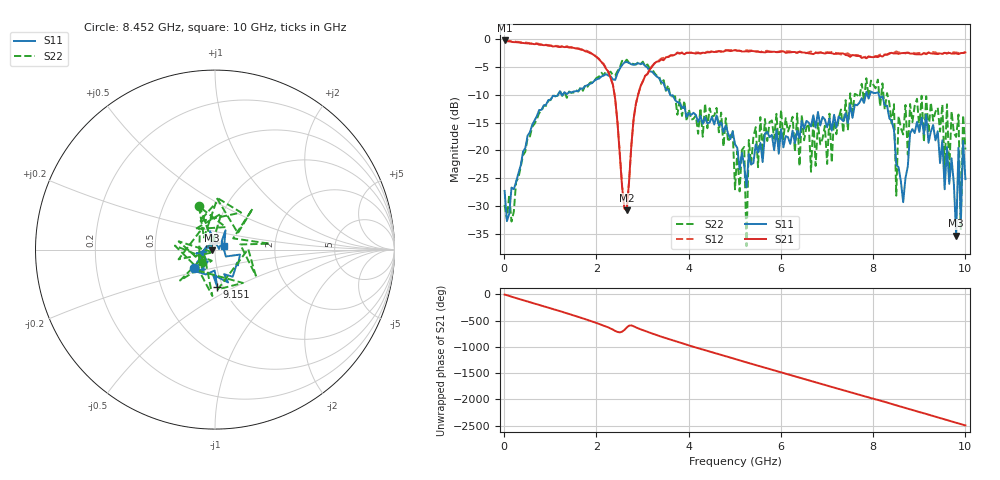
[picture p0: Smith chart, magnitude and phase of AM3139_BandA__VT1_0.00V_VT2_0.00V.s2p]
! Date/Time: Tue, Nov 13, 2018 4:56 PM
! Network Analyzer: Agilent Technologies E8364B Rev: A.07.50.67
! Sweep from 0.010 to 10.000 GHz, 201 Points, Sweep Type: LIN
! Power Supply: -0.000 V, 0.000 A
# Hz S DB R 50
!freq MagS11 AngS11 MagS21 AngS21 MagS12 AngS12 MagS22 AngS22
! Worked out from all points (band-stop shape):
!   201 points, 10 MHz to 10 GHz, reference 50 ohm
!   highest |S21| = -0.20 dB at 10 MHz (marker M1); lowest = -30.8 dB at 2.657 GHz (marker M2)
!   |S21| within 3 dB of the highest: start of sweep to 2.004 GHz; 3.537 GHz to 7.732 GHz (4.195 GHz wide, 74.4 % of centre)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
!   lowest |S11| = -35.4 dB at 9.8 GHz (marker M3), VSWR 1.03, Z = 48.4 - j0.4 ohm
!   |S11| at or under -10 dB: start of sweep to 1.167 GHz; 3.601 GHz to 7.839 GHz (4.239 GHz wide, 74.1 % of centre); 8.124 GHz to end of sweep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
!   |S22| runs from -37.3 to -3.7 dB; largest |S21 - S12| = 0.035
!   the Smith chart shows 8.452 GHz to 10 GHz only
!   S11 on the Smith chart (normalised r, x): 8.452 GHz: 0.78, -0.16; 9.151 GHz: 0.94, -0.41; 10 GHz: 1.11, +0.04
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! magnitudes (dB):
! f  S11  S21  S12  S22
! 10 MHz  -27.3  -0.2  -0.2  -29.8
! 1.708 GHz  -8.9  -1.9  -1.8  -9.3
! 2.358 GHz  -7.2  -8.2  -8.2  -6.5
! 2.657 GHz  -4.1  -30.8  -30.8  -3.7
! 2.857 GHz  -4.4  -11.6  -11.6  -4.6
! 3.357 GHz  -7.0  -4.0  -3.8  -6.5
! 5.005 GHz  -18.9  -1.9  -2.0  -27.0
! 5.205 GHz  -22.8  -2.2  -2.0  -19.4
! 5.255 GHz  -26.7  -2.1  -2.0  -37.3
! 5.305 GHz  -20.7  -2.2  -2.0  -18.1
! 5.554 GHz  -18.7  -2.3  -2.3  -14.0
! 6.703 GHz  -13.7  -2.7  -2.4  -14.2
! 8.352 GHz  -14.2  -2.5  -2.6  -11.5
! 8.452 GHz  -16.3  -2.6  -2.4  -11.7
! 8.501 GHz  -22.6  -2.5  -2.2  -28.2
! 8.551 GHz  -23.0  -2.6  -2.4  -13.8
! 9.151 GHz  -13.6  -2.6  -2.7  -10.3
! 9.8 GHz  -35.4  -2.6  -2.4  -17.6
! 9.85 GHz  -19.5  -2.7  -2.5  -13.6
! 9.9 GHz  -32.9  -2.5  -2.4  -34.4
! 9.95 GHz  -18.3  -2.5  -2.5  -13.7
! 10 GHz  -25.2  -2.4  -2.3  -19.9
